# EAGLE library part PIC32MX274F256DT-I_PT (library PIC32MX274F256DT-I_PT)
32-bit Microcontrollers - MCU 256KB Flash, 64KB RAM, 10-Bit ADC, UART, SPI/I2S, I2C + VBATT Pin, USB Source: Datasheet
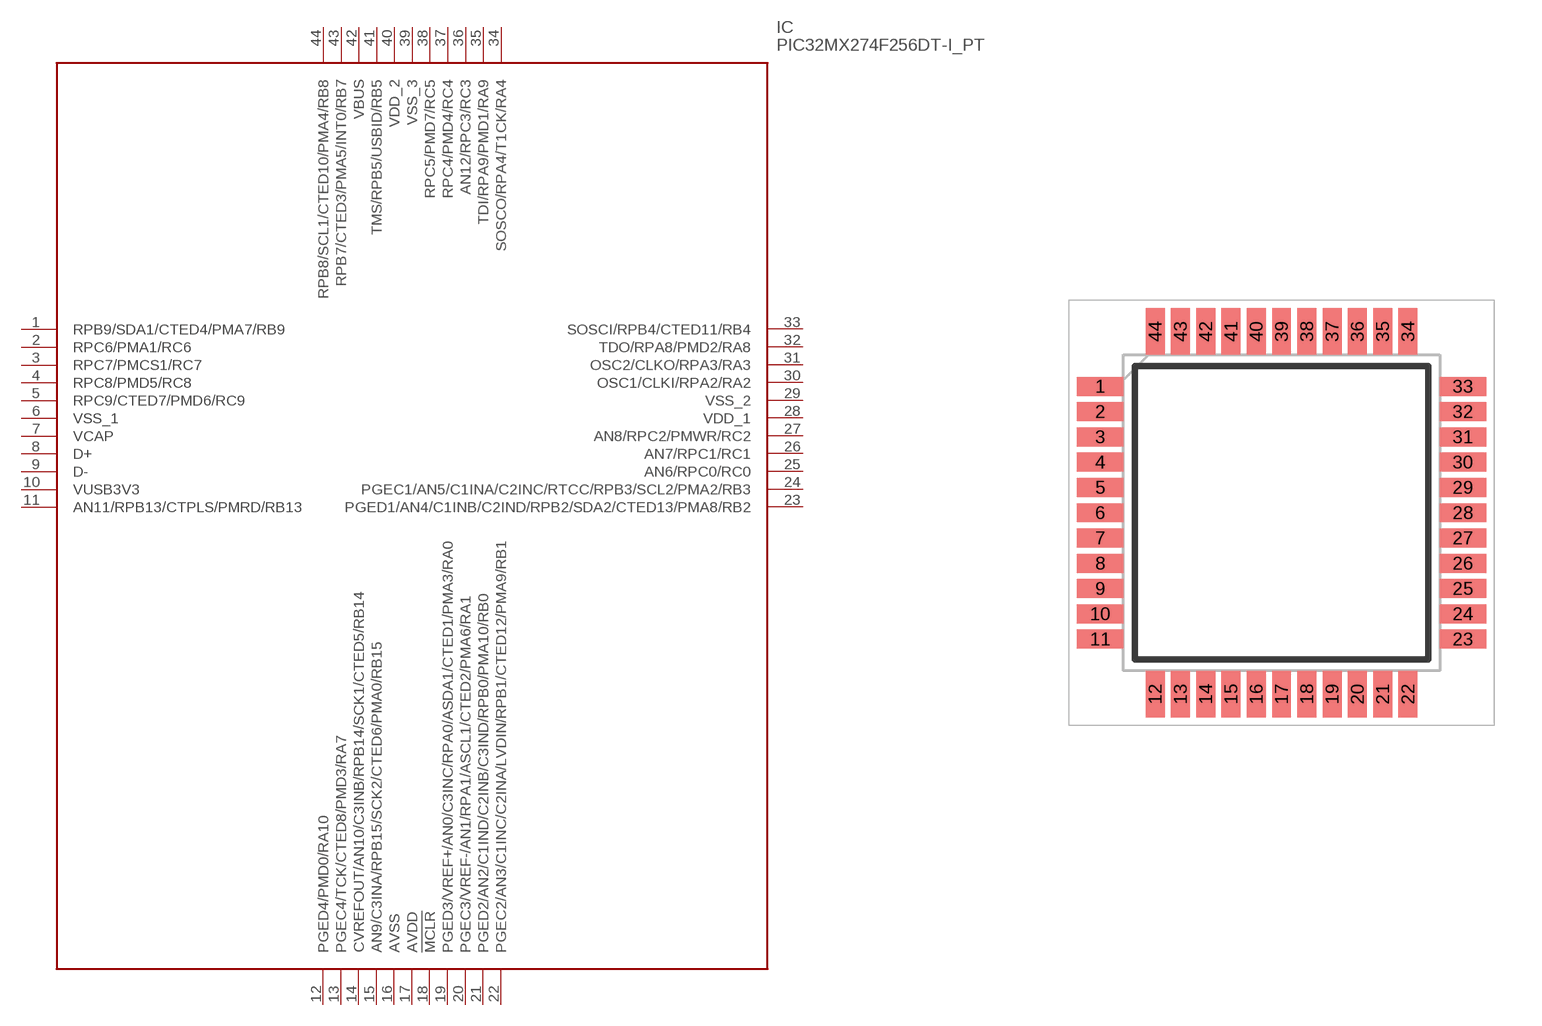
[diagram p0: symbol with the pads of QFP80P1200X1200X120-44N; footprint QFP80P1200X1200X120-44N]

Designator prefix IC

## PIC32MX274F256DT-I_PT (Arrow_Part_Number: PIC32MX274F256DT-I/PT; Description: 32-bit Microcontrollers - MCU 256KB Flash, 64KB RAM, 10-Bit ADC, UART, SPI/I2S, I2C + VBATT Pin, USB; Height: 1.2mm; Manufacturer_Name: Microchip; Manufacturer_Part_Number: PIC32MX274F256DT-I/PT)  [QFP80P1200X1200X120-44N]
1  RPB9/SDA1/CTED4/PMA7/RB9
2  RPC6/PMA1/RC6
3  RPC7/PMCS1/RC7
4  RPC8/PMD5/RC8
5  RPC9/CTED7/PMD6/RC9
6  VSS_1
7  VCAP
8  D+
9  D-
10  VUSB3V3
11  AN11/RPB13/CTPLS/PMRD/RB13
12  PGED4/PMD0/RA10
13  PGEC4/TCK/CTED8/PMD3/RA7
14  CVREFOUT/AN10/C3INB/RPB14/SCK1/CTED5/RB14
15  AN9/C3INA/RPB15/SCK2/CTED6/PMA0/RB15
16  AVSS
17  AVDD
18  !MCLR
19  PGED3/VREF+/AN0/C3INC/RPA0/ASDA1/CTED1/PMA3/RA0
20  PGEC3/VREF-/AN1/RPA1/ASCL1/CTED2/PMA6/RA1
21  PGED2/AN2/C1IND/C2INB/C3IND/RPB0/PMA10/RB0
22  PGEC2/AN3/C1INC/C2INA/LVDIN/RPB1/CTED12/PMA9/RB1
23  PGED1/AN4/C1INB/C2IND/RPB2/SDA2/CTED13/PMA8/RB2
24  PGEC1/AN5/C1INA/C2INC/RTCC/RPB3/SCL2/PMA2/RB3
25  AN6/RPC0/RC0
26  AN7/RPC1/RC1
27  AN8/RPC2/PMWR/RC2
28  VDD_1
29  VSS_2
30  OSC1/CLKI/RPA2/RA2
31  OSC2/CLKO/RPA3/RA3
32  TDO/RPA8/PMD2/RA8
33  SOSCI/RPB4/CTED11/RB4
34  SOSCO/RPA4/T1CK/RA4
35  TDI/RPA9/PMD1/RA9
36  AN12/RPC3/RC3
37  RPC4/PMD4/RC4
38  RPC5/PMD7/RC5
39  VSS_3
40  VDD_2
41  TMS/RPB5/USBID/RB5
42  VBUS
43  RPB7/CTED3/PMA5/INT0/RB7
44  RPB8/SCL1/CTED10/PMA4/RB8

## Footprint QFP80P1200X1200X120-44N (pad centres in mm)
(PT)44-Lead(TQFP)
smd 1.475 x 0.6: 1 -5.738,4; 2 -5.738,3.2; 3 -5.738,2.4; 4 -5.738,1.6; 5 -5.738,0.8; 6 -5.738,0; 7 -5.738,-0.8; 8 -5.738,-1.6; 9 -5.738,-2.4; 10 -5.738,-3.2; 11 -5.738,-4; 23 5.738,-4; 24 5.738,-3.2; 25 5.738,-2.4; 26 5.738,-1.6; 27 5.738,-0.8; 28 5.738,0; 29 5.738,0.8; 30 5.738,1.6; 31 5.738,2.4; 32 5.738,3.2; 33 5.738,4
smd 0.6 x 1.475: 12 -4,-5.738; 13 -3.2,-5.738; 14 -2.4,-5.738; 15 -1.6,-5.738; 16 -0.8,-5.738; 17 0,-5.738; 18 0.8,-5.738; 19 1.6,-5.738; 20 2.4,-5.738; 21 3.2,-5.738; 22 4,-5.738; 34 4,5.738; 35 3.2,5.738; 36 2.4,5.738; 37 1.6,5.738; 38 0.8,5.738; 39 0,5.738; 40 -0.8,5.738; 41 -1.6,5.738; 42 -2.4,5.738; 43 -3.2,5.738; 44 -4,5.738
